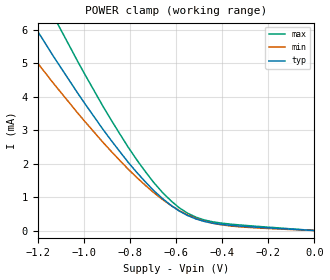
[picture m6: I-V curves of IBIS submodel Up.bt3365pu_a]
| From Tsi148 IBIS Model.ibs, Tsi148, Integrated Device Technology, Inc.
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[Submodel]  Up.bt3365pu_a
Submodel_type   Dynamic_clamp
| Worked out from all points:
|   POWER clamp passes 1 mA (typ) near -0.67 V on its own axis
[POWER Clamp]   | Note: Vtable = Vcc - Vout
| Voltage   I(typ)   I(min)   I(max)
-3.6V     35.64mA    28.8mA     43.89mA
-1.32V    7.295mA    6.083mA    8.995mA
-1.283V   6.881mA    5.75mA     8.484mA
-1.21V    6.066mA    5.094mA    7.477mA
-1.1V     4.877mA    4.135mA    6.009mA
-917mV    3.026mA    2.638mA    3.716mA
-807mV    2.036mA    1.831mA    2.486mA
-697mV    1.196mA    1.134mA    1.438mA
-587mV    586uA      599uA      683uA
-513mV    344uA      359uA      397uA
-440mV    218uA      215uA      259uA
0V        1uA        1uA        2uA
